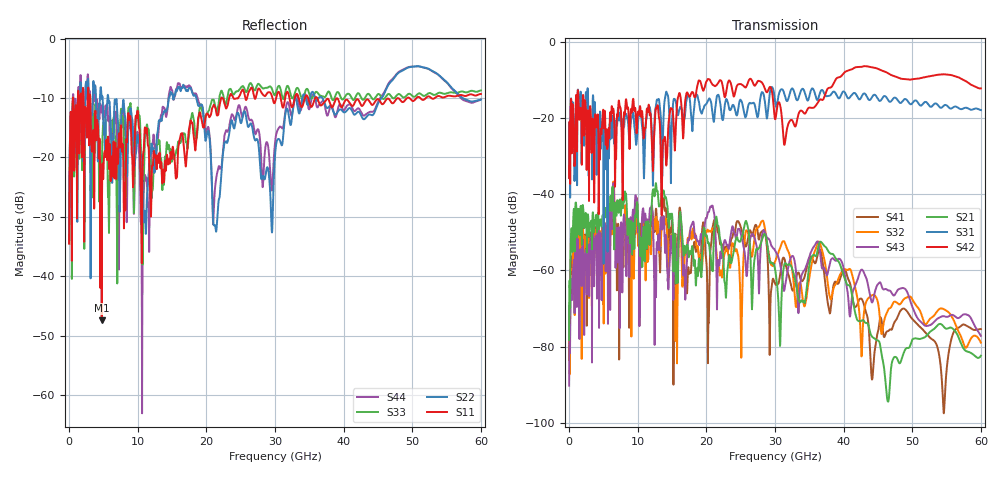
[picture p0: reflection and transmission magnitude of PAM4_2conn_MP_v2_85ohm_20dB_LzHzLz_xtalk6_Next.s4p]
! Info: Touchstone file created by Circ.  Input file=FAB50GbE_2conn_Midplane_Examax_Topo2_v2_85ohm_20dB_LzHzLz.circ
# Hz S RI R 50
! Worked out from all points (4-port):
!   6000 points, 10 MHz to 60 GHz, reference 50 ohm
!   strongest paths, dB at 10 MHz, 15.01 GHz, 30.01 GHz, 45.01 GHz, 60 GHz:
!     S42: -35.6, -17.4, -20.2, -7.0, -12.1
!     S31: -35.7, -20.5, -15.4, -14.9, -17.8
!     S21: -78.3, -45.3, -59.6, -78.4, -82.4
!     S43: -90.3, -53.3, -54.7, -63.6, -77.2
!     S32: -78.9, -51.1, -57.7, -68.5, -79.0
!     S41: -83.6, -47.1, -63.4, -76.1, -75.4
!   lowest |S11| = -47.4 dB at 4.76 GHz (marker M1), VSWR 1.01, Z = 49.6 - j0.173 ohm
!   |S11| at or under -10 dB: 3.09 GHz to 22.16 GHz (19.07 GHz wide, 151 % of centre); 34.83 GHz to 35.87 GHz (1.045 GHz wide, 2.96 % of centre); 36.15 GHz to 49.26 GHz (13.11 GHz wide, 30.7 % of centre)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
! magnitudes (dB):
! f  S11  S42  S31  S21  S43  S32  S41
! 10 MHz  -34.5  -35.6  -35.7  -78.3  -90.3  -78.9  -83.6
! 830 MHz  -16.6  -31.7  -30.2  -55.0  -63.3  -64.4  -60.9
! 4.76 GHz  -47.4  -22.9  -22.1  -48.4  -66.9  -59.4  -57.0
! 10.65 GHz  -29.4  -18.2  -22.1  -58.9  -45.5  -47.2  -47.0
! 15.93 GHz  -18.3  -14.1  -18.8  -53.9  -51.6  -55.0  -48.8
! 21.29 GHz  -11.6  -11.5  -17.5  -47.7  -48.7  -51.4  -46.3
! 60 GHz  -9.3  -12.1  -17.8  -82.4  -77.2  -79.0  -75.4
